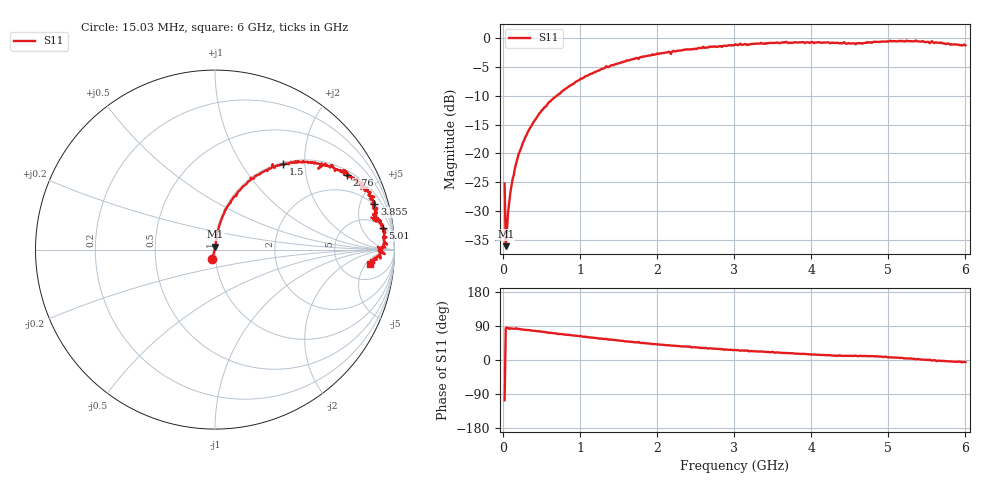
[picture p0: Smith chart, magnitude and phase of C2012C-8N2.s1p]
!	Network	Analyzer	HP8753E.07.74:	Oct	30	2002	Serial	No.	JP38451487
!	Hewlett-Packard
!	7	Sep	2009	10:43:13
!	Frequency	S11
#	HZ	S	RI	R	50
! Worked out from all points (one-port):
!   400 points, 15.03 MHz to 6 GHz, reference 50 ohm
!   lowest |S11| = -36.1 dB at 30.03 MHz (marker M1), VSWR 1.03, Z = 50.1 + j1.55 ohm
!   |S11| at or under -10 dB: start of sweep to 689.7 MHz
!   S11 on the Smith chart (normalised r, x): 15.03 MHz: 0.96, -0.10; 1.5 GHz: 1.03, +1.56; 2.76 GHz: 1.16, +3.43; 3.855 GHz: 1.92, +6.57; 5.01 GHz: 6, +13; 6 GHz: 10, -7
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1.502992e7  -0.0152 -0.0525
3.002985e7  0.00171 0.0155
6.00297e7  0.00308 0.0306
9.002955e7  0.00511 0.0452
1.95029e8  0.0132 0.0967
3.150284e8  0.0292 0.15
4.650277e8  0.0533 0.216
7.650262e8  0.128 0.323
1.335023e9  0.321 0.476
1.500022e9  0.381 0.475
1.515022e9  0.385 0.473
2.265019e9  0.624 0.472
2.760016e9  0.737 0.417
3.015015e9  0.798 0.394
3.165014e9  0.788 0.376
3.195014e9  0.815 0.338
3.495013e9  0.847 0.337
3.525012e9  0.863 0.297
3.765011e9  0.873 0.278
3.855011e9  0.887 0.254
4.515007e9  0.886 0.172
5.010005e9  0.936 0.121
5.265004e9  0.946 0.0639
5.535002e9  0.907 0.0152
5.565002e9  0.946 -0.0254
5.595002e9  0.911 -0.00348
5.625002e9  0.922 -0.05
6e9  0.865 -0.0801
